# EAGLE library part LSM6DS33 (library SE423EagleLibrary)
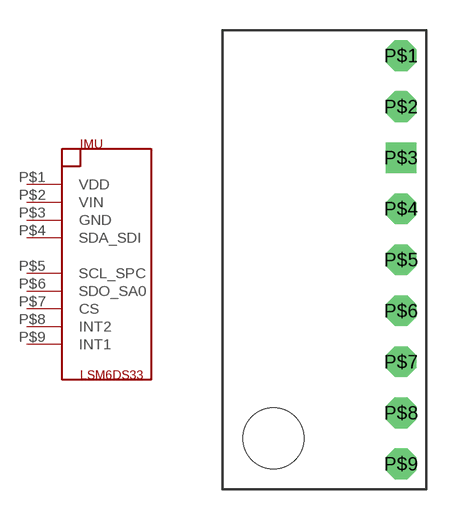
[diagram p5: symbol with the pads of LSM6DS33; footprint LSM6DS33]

Designator prefix IMU

## LSM6DS33  [LSM6DS33]
P$1  VDD
P$2  VIN
P$3  GND
P$4  SDA_SDI
P$5  SCL_SPC
P$6  SDO_SA0
P$7  CS
P$8  INT2
P$9  INT1

## Footprint LSM6DS33 (pad centres in mm)
drill 1.016 octagon: P$1 0,5.08; P$2 0,2.54; P$4 0,-2.54; P$5 0,-5.08; P$6 0,-7.62; P$7 0,-10.16; P$8 0,-12.7; P$9 0,-15.24
drill 1.016 square: P$3 0,0
hole 3.048 at -6.35,-13.97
